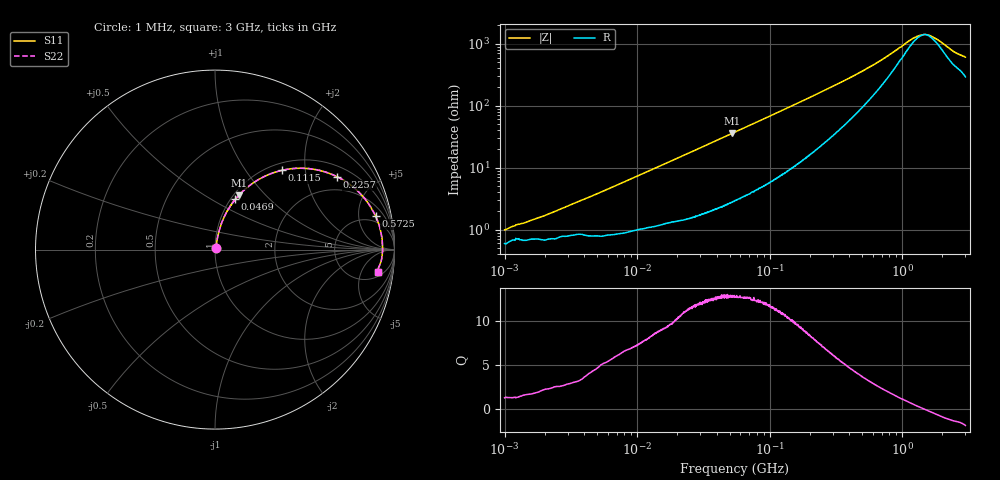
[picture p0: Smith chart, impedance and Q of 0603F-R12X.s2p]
!s-Parameter Generated by FASTRON Sdn. Bhd.
!FASTRON P/N : 0603F-R12X
!Keysight Technologies: E4991B_MY54100416_A.01.15
!Date: Thu Jun 20 13:06:03 2024
!Version  :Rev00  Thu Jun 20 13:06:03 2024
!Data & Calibration Information:
!Freq  S11  S21  S12  S22
!PortZ  Port1:50+j0  Port2:50+j0
!When reading reference impedance value at option line is always used.
! Remarks : This data is being provided solely for informational purposes.
# Hz S dB R 50
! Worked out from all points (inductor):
!   1601 points, 1 MHz to 3 GHz, reference 50 ohm
!   read as one part in series: L = 120 nH near 3.225 MHz
!   highest Q = 12.9 at 52.1 MHz (marker M1), where L = 109 nH
!   self-resonance near 1.484 GHz
!   S11 on the Smith chart (normalised r, x): 1 MHz: 1.01, +0.02; 46.9 MHz: 1.05, +0.65; 111.5 MHz: 1.13, +1.51; 225.7 MHz: 1.40, +3.04; 572.5 MHz: 3.58, +8.12; 3 GHz: 7, -11
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1000000  -40.10 52.5  -0.05 -0.5  -0.05 -0.5  -40.10 52.5
2035141  -35.40 65.6  -0.06 -0.9  -0.06 -0.9  -35.40 65.6
3804036  -30.60 72.0  -0.08 -1.6  -0.08 -1.6  -30.60 72.0
1.447069e7  -19.80 77.7  -0.15 -5.8  -0.15 -5.8  -19.80 77.7
2.815302e7  -14.40 74.3  -0.30 -10.9  -0.30 -10.9  -14.40 74.3
4.6902e7  -10.40 68.1  -0.63 -17.5  -0.63 -17.5  -10.40 68.1
5.209891e7  -9.65 66.4  -0.73 -19.2  -0.73 -19.2  -9.65 66.4
5.504702e7  -9.24 65.4  -0.80 -20.1  -0.80 -20.1  -9.24 65.4
7.774719e7  -6.87 58.5  -1.36 -26.9  -1.36 -26.9  -6.87 58.5
1.114693e8  -4.74 49.7  -2.32 -35.2  -2.32 -35.2  -4.74 49.7
1.520175e8  -3.30 41.4  -3.55 -42.9  -3.55 -42.9  -3.30 41.4
2.083556e8  -2.23 32.9  -5.24 -50.1  -5.24 -50.1  -2.23 32.9
2.257233e8  -2.02 30.8  -5.74 -51.8  -5.74 -51.8  -2.02 30.8
3.50605e8  -1.21 20.6  -8.92 -58.8  -8.92 -58.8  -1.21 20.6
5.725215e8  -0.78 11.8  -13.40 -60.6  -13.40 -60.6  -0.78 11.8
7.925923e8  -0.66 7.2  -17.00 -55.6  -17.00 -55.6  -0.66 7.2
1.206698e9  -0.60 2.2  -22.30 -28.5  -22.30 -28.5  -0.60 2.2
1.360679e9  -0.60 0.9  -23.30 -13.1  -23.30 -13.1  -0.60 0.9
1.496395e9  -0.60 -0.1  -23.60 1.3  -23.60 1.3  -0.60 -0.1
1.791767e9  -0.62 -2.0  -22.30 25.7  -22.30 25.7  -0.62 -2.0
2.443543e9  -0.72 -5.6  -18.20 46.9  -18.20 46.9  -0.72 -5.6
3e9  -0.74 -7.6  -16.40 53.6  -16.40 53.6  -0.74 -7.6
